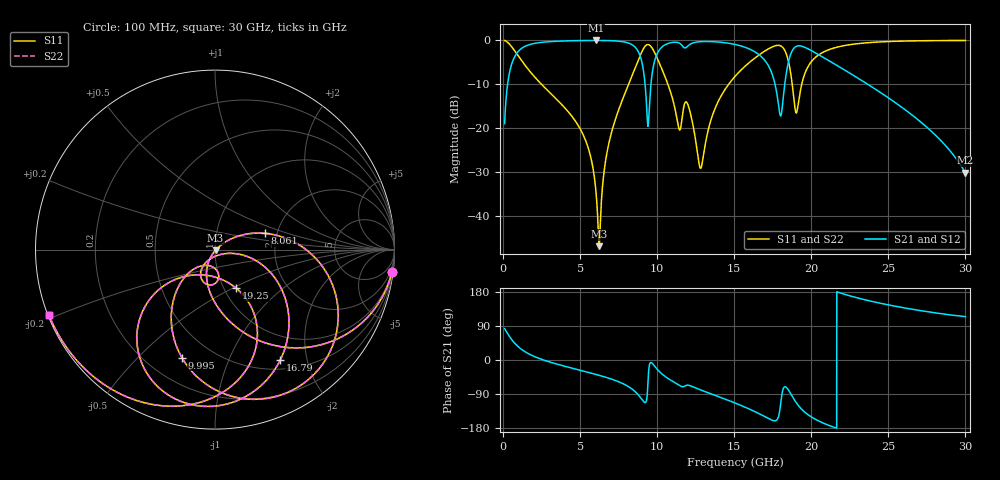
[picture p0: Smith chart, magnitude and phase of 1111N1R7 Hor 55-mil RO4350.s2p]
# GHz S MA R 50
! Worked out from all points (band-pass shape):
!   3201 points, 100 MHz to 30 GHz, reference 50 ohm
!   highest |S21| = -0.04 dB at 6.024 GHz (marker M1); lowest = -30.1 dB at 30 GHz (marker M2)
!   |S21| within 3 dB of the highest: 871.4 MHz to 8.838 GHz (7.966 GHz wide, 164 % of centre); 10 GHz to 16.52 GHz (6.522 GHz wide, 49.2 % of centre)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
!   lowest |S11| = -46.8 dB at 6.229 GHz (marker M3), VSWR 1.01, Z = 50.3 - j0.33 ohm
!   |S11| at or under -10 dB: 2.492 GHz to 8.145 GHz (5.653 GHz wide, 106 % of centre); 10.69 GHz to 14.64 GHz (3.945 GHz wide, 31.1 % of centre); 18.76 GHz to 19.38 GHz (615.1 MHz wide, 3.23 % of centre)
!   |S22| runs from -46.8 to 0.0 dB; largest |S21 - S12| = 0
!   S11 on the Smith chart (normalised r, x): 100 MHz: 1, -16; 8.061 GHz: 1.72, +0.34; 9.995 GHz: 0.34, -0.68; 16.79 GHz: 0.62, -1.57; 19.25 GHz: 1.14, -0.52; 30 GHz: 0.00, -0.19
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0.1  0.9936 -7.1  0.1127 82.8  0.1127 82.8  0.9936 -7.1
1.07175  0.6317 -57.9  0.7741 32.0  0.7741 32.0  0.6317 -57.9
5.089563  0.09222 -116.0  0.992 -28.0  0.992 -28.0  0.09222 -116.0
6.023937  0.01942 -115.5  0.9949 -38.0  0.9949 -38.0  0.01942 -115.5
6.2295  0.00457 -45.9  0.9947 -40.3  0.9947 -40.3  0.00457 -45.9
6.8275  0.06288 36.8  0.9912 -47.6  0.9912 -47.6  0.06288 36.8
8.060875  0.2906 18.2  0.9387 -68.4  0.9387 -68.4  0.2906 18.2
8.911156  0.6795 -16.3  0.6506 -98.9  0.6506 -98.9  0.6795 -16.3
9.397031  0.8945 -58.8  0.1048 -64.2  0.1048 -64.2  0.8945 -58.8
9.995031  0.6297 -107.0  0.7016 -24.1  0.7016 -24.1  0.6297 -107.0
10.06978  0.588 -110.9  0.7436 -27.5  0.7436 -27.5  0.588 -110.9
11.41528  0.09835 -116.3  0.9324 -66.6  0.9324 -66.6  0.09835 -116.3
12.00394  0.1833 -113.4  0.8646 -66.4  0.8646 -66.4  0.1833 -113.4
12.81684  0.035 -69.7  0.9641 -79.0  0.9641 -79.0  0.035 -69.7
15.05  0.3881 -26.9  0.8964 -113.4  0.8964 -113.4  0.3881 -26.9
16.78794  0.7155 -59.5  0.644 -145.2  0.644 -145.2  0.7155 -59.5
18.00262  0.8644 -103.6  0.1379 -118.8  0.1379 -118.8  0.8644 -103.6
18.49784  0.5941 -135.9  0.5472 -77.8  0.5472 -77.8  0.5941 -135.9
19.25469  0.2461 -61.1  0.8636 -124.7  0.8636 -124.7  0.2461 -61.1
20.03956  0.5811 -66.7  0.7575 -151.1  0.7575 -151.1  0.5811 -66.7
25.01978  0.9673 -126.1  0.2207 145.3  0.2207 145.3  0.9673 -126.1
30  0.9948 -158.6  0.03117 114.4  0.03117 114.4  0.9948 -158.6
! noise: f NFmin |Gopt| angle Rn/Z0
0.1  0.001939  0.9171  2.97  0.005156
3.417  0.01192  0.5534  24.88  0.004572
6.743  0.02676  0.6033  43.12  0.01087
10.06  0.1244  0.8572  63.74  0.1347
13.39  0.07709  0.7214  81.4  0.03214
16.7  0.1431  0.809  97.78  0.06847
20.03  0.1542  0.7911  114.5  0.04604
23.35  0.173  0.803  127.2  0.03786
26.67  0.3291  0.8928  142.8  0.07001
30  1.227  0.9708  159.3  0.3153
